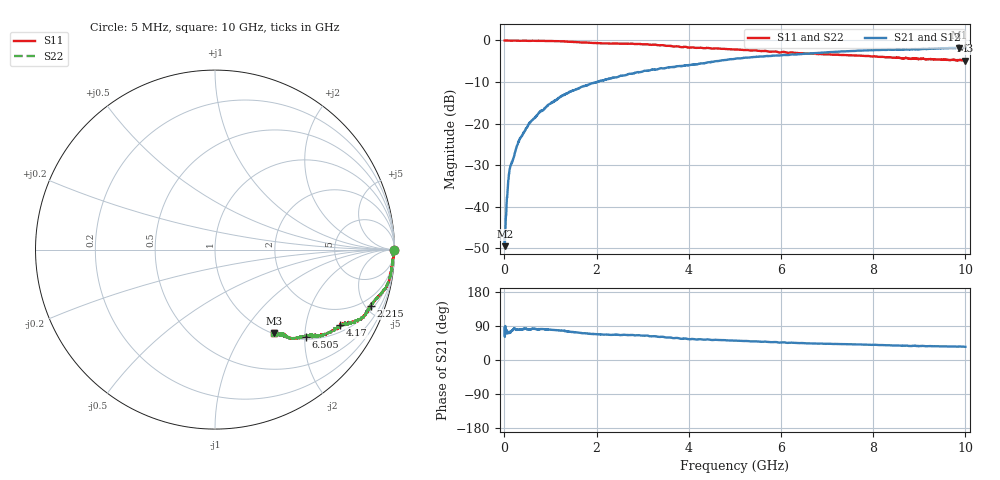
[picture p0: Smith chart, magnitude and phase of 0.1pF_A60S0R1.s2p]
! Amotech Co.,Ltd.
! http://www.amotech.co.kr/
! Part Number: A60S0R1
! These Parameters are Measured in Series Mode Connection
! Operation Temp=25[degC], DC Bias Voltage=0[V]
! Freq. Start=5[MHz] Stop=10[GHz], 2000[Steps]
! Date: Monday, July 13, 2020, 01:23:14
# GHZ S RI R 50.000000
!Freq.(Hz) S11(Real) S11(Imag) S21(Real) S21(Imag) S12(Real) S12(Imag) S22(Real) S22(Imag)
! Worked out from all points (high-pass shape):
!   2000 points, 5 MHz to 10 GHz, reference 50 ohm
!   highest |S21| = -1.75 dB at 9.865 GHz (marker M1); lowest = -49.5 dB at 10 MHz (marker M2)
!   |S21| within 3 dB of the highest: 4.755 GHz to end of sweep
!   lowest |S11| = -4.9 dB at 10 GHz (marker M3), VSWR 3.66, Z = 50.7 - j70 ohm
!   |S11| at or under -10 dB: nowhere
!   |S22| runs from -4.9 to 0.0 dB; largest |S21 - S12| = 1.4e-15
!   S11 on the Smith chart (normalised r, x): 5 MHz: open; 2.215 GHz: 1.30, -5.40; 4.17 GHz: 1.26, -3.13; 6.505 GHz: 1.06, -2.02; 10 GHz: 1.01, -1.40
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0.005  0.9996 -0.00494  0.000432 0.00494  0.000432 0.00494  0.9996 -0.00494
0.01  0.9984 -0.00293  0.00162 0.00293  0.00162 0.00293  0.9984 -0.00293
0.04  0.9973 -0.00743  0.00271 0.00743  0.00271 0.00743  0.9973 -0.00743
0.08  0.9943 -0.0175  0.00565 0.0175  0.00565 0.0175  0.9943 -0.0175
0.095  0.9937 -0.0227  0.00633 0.0227  0.00633 0.0227  0.9937 -0.0227
0.125  0.9916 -0.0284  0.00841 0.0284  0.00841 0.0284  0.9916 -0.0284
0.16  0.9922 -0.0337  0.00778 0.0337  0.00778 0.0337  0.9922 -0.0337
0.265  0.991 -0.0509  0.00897 0.0509  0.00897 0.0509  0.991 -0.0509
0.35  0.9887 -0.0664  0.0113 0.0664  0.0113 0.0664  0.9887 -0.0664
0.56  0.9838 -0.1022  0.0162 0.1022  0.0162 0.1022  0.9838 -0.1022
0.94  0.9712 -0.1637  0.0288 0.1637  0.0288 0.1637  0.9712 -0.1637
1.245  0.9544 -0.2092  0.0456 0.2092  0.0456 0.2092  0.9544 -0.2092
1.675  0.9106 -0.2615  0.0894 0.2615  0.0894 0.2615  0.9106 -0.2615
2.215  0.8667 -0.3135  0.1333 0.3135  0.1333 0.3135  0.8667 -0.3135
3.34  0.7811 -0.3969  0.2189 0.3969  0.2189 0.3969  0.7811 -0.3969
4.17  0.6969 -0.4198  0.3031 0.4198  0.3031 0.4198  0.6969 -0.4198
5.005  0.6202 -0.4682  0.3798 0.4682  0.3798 0.4682  0.6202 -0.4682
6.505  0.5058 -0.4847  0.4942 0.4847  0.4942 0.4847  0.5058 -0.4847
6.67  0.4951 -0.487  0.5049 0.487  0.5049 0.487  0.4951 -0.487
8.335  0.3977 -0.4873  0.6023 0.4873  0.6023 0.4873  0.3977 -0.4873
9.865  0.3339 -0.4743  0.6661 0.4743  0.6661 0.4743  0.3339 -0.4743
10  0.3302 -0.4656  0.6698 0.4656  0.6698 0.4656  0.3302 -0.4656
